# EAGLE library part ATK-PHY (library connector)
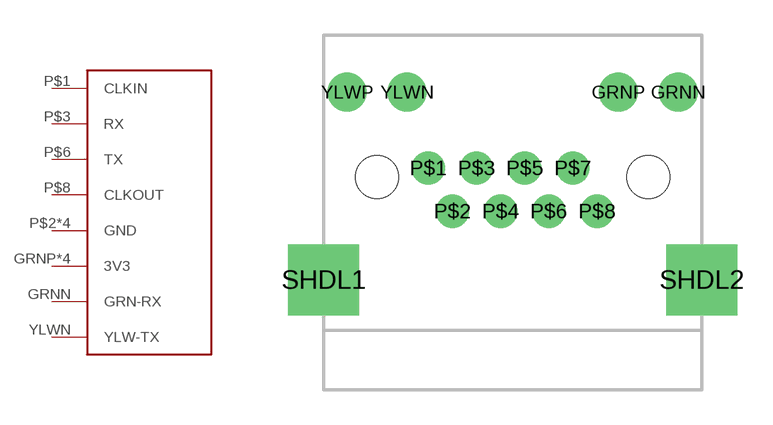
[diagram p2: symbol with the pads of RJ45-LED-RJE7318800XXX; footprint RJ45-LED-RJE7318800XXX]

Designator prefix J

## ATK-PHY  [RJ45-LED-RJE7318800XXX]
GRNN  GRN-RX
GRNP  3V3
P$1  CLKIN
P$2  GND
P$3  RX
P$4  3V3
P$5  3V3
P$6  TX
P$7  GND
P$8  CLKOUT
SHDL1  GND
SHDL2  GND
YLWN  YLW-TX
YLWP  3V3

## Footprint RJ45-LED-RJE7318800XXX (pad centres in mm)
drill 1.1: GRNN 7.01,3.6; GRNP 4.47,3.6; YLWN -4.47,3.6; YLWP -7.01,3.6
drill 0.9: P$1 -3.57,0.38; P$2 -2.55,-1.45; P$3 -1.53,0.38; P$4 -0.51,-1.45; P$5 0.51,0.38; P$6 1.53,-1.45; P$7 2.55,0.38; P$8 3.57,-1.45
drill 2 square: SHDL1 -8,-4.35; SHDL2 8,-4.35
hole 1.8 at -5.74,0
hole 1.8 at 5.74,0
